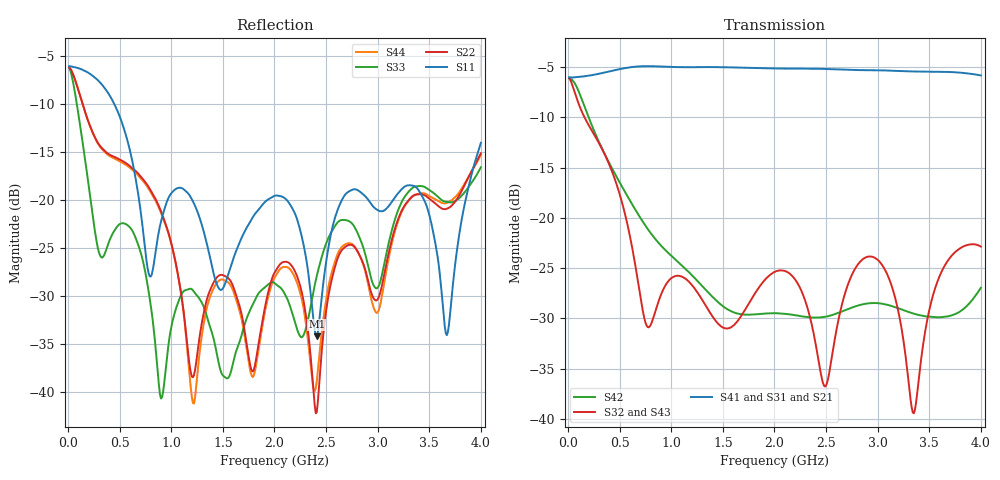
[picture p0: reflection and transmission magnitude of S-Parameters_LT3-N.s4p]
! MTS Systemtechnik GmbH
! S-Parameters
! Model: z.B.: LT3-588P-4G
! Rohde & Schwarz ZVB8 2Ports - Version 3.20 - 1145.1010k08 SN: 100119
! Converted & adapted with MATLAB
!  OUT 3 (Port 4)
!  o
!		|  MTS  |
! C (Port 1) o--| LT3-588P-4G |--o OUT 2 (Port 3)
!  o
!  OUT 1 (Port 2)
! S4P File: Measurements:
! <S11,S12,S13,S14>,
! <S21,S22,S23,S24>,
! <S31,S32,S33,S34>,
! <S41,S42,S43,S44>:
# HZ  S  DB  R  50.00
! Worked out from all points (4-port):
!   400 points, 10 MHz to 4 GHz, reference 50 ohm
!   strongest paths, dB at 10 MHz, 1.01 GHz, 2.01 GHz, 3.01 GHz, 4 GHz:
!     S41: -6.0, -5.0, -5.1, -5.3, -5.8
!     S31: -6.0, -5.0, -5.2, -5.3, -5.8
!     S21: -6.0, -5.0, -5.2, -5.4, -5.9
!     S32: -6.1, -25.9, -25.3, -24.3, -22.9
!     S43: -6.1, -25.8, -25.5, -24.3, -23.0
!     S42: -6.1, -23.9, -29.5, -28.5, -27.0
!   lowest |S11| = -34.2 dB at 2.41 GHz (marker M1), VSWR 1.04, Z = 49.1 - j1.7 ohm
!   |S11| at or under -10 dB: 447.4 MHz to end of sweep
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1e7  -6.05 177.7  -6.02 -2.6  -6.02 -2.6  -6.02 -2.6
     -6.03 -2.6  -6.18 171.1  -6.11 -5.7  -6.07 -6.1
     -6.03 -2.6  -6.12 -5.7  -6.22 171.5  -6.11 -5.7
     -6.03 -2.6  -6.08 -6.1  -6.12 -5.7  -6.18 171.1
9e8  -22.26 160.1  -5.00 106.0  -4.97 106.0  -4.94 106.0
     -5.00 106.0  -21.17 151.1  -27.64 -113.9  -22.75 -56.3
     -4.97 106.0  -27.65 -113.8  -40.70 120.9  -27.48 -112.9
     -4.95 106.0  -22.76 -56.3  -27.49 -112.9  -21.33 150.2
1.57e9  -27.15 151.9  -5.08 -86.0  -5.05 -86.0  -5.03 -86.0
        -5.08 -86.0  -28.37 174.9  -30.93 -159.7  -29.25 -19.1
        -5.06 -86.0  -30.94 -159.7  -38.18 -30.2  -30.95 -159.8
        -5.03 -86.0  -29.24 -19.0  -30.95 -159.7  -28.82 177.8
2.41e9  -34.21 -117.2  -5.21 32.5  -5.18 32.6  -5.16 32.5
        -5.22 32.5  -42.11 -125.0  -33.18 100.8  -29.92 -39.0
        -5.19 32.7  -33.19 100.9  -27.92 -88.2  -33.71 102.1
        -5.17 32.5  -29.93 -39.0  -33.73 102.2  -38.87 -110.5
3.12e9  -20.45 -157.2  -5.40 -174.1  -5.35 -173.6  -5.35 -174.1
        -5.40 -174.1  -24.89 -83.1  -26.31 43.5  -28.73 -16.7
        -5.35 -173.6  -26.32 43.6  -23.89 -92.4  -26.36 44.7
        -5.36 -174.1  -28.73 -16.7  -26.36 44.7  -25.35 -78.9
3.67e9  -34.10 139.0  -5.51 22.7  -5.44 23.6  -5.46 22.9
        -5.53 22.7  -20.91 -112.9  -24.40 60.4  -29.81 91.8
        -5.45 23.6  -24.41 60.5  -20.20 -129.2  -24.53 60.8
        -5.48 22.9  -29.82 91.8  -24.55 60.8  -20.30 -112.9
4e9  -14.04 79.4  -5.87 -79.0  -5.77 -77.7  -5.81 -78.7
     -5.91 -79.0  -15.13 -102.5  -22.84 -14.6  -26.92 -33.6
     -5.79 -77.7  -22.87 -14.5  -16.59 -112.5  -23.00 -13.0
     -5.84 -78.7  -26.96 -33.4  -23.03 -12.9  -15.31 -104.2
